{attribute 'qualified_only'}
{attribute 'strict'}
TYPE E_PTP_PORT_STATE :
(
	INVALID := 0,
	PTP_INITIALISZING:=1,
	PTP_FAULTY:=2,
	PTP_DISABLED:=3,
	PTP_LISTENING:=4,
	PTP_PRE_MASTER:=5,
	PTP_MASTER:=6,
	PTP_PASSIVE:=7,
	PTP_UNCALIBRATED:=8,
	PTP_SLAVE:=9
);
END_TYPE
